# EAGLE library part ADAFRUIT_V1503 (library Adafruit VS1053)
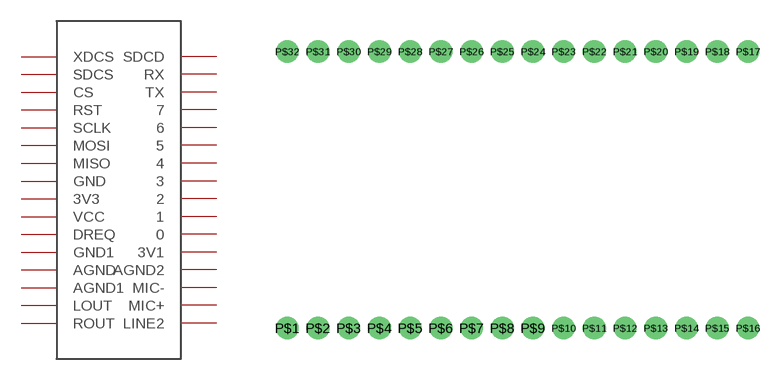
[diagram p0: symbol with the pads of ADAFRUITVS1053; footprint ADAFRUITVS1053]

Designator prefix -

## ADAFRUIT_V1503  [ADAFRUITVS1053]
P$1  XDCS
P$2  SDCS
P$3  CS
P$4  RST
P$5  SCLK
P$6  MOSI
P$7  MISO
P$8  GND
P$9  3V3
P$10  VCC
P$11  DREQ
P$12  GND1
P$13  AGND
P$14  AGND1
P$15  LOUT
P$16  ROUT
P$17  LINE2
P$18  MIC+
P$19  MIC-
P$20  AGND2
P$21  3V1
P$22  0
P$23  1
P$24  2
P$25  3
P$26  4
P$27  5
P$28  6
P$29  7
P$30  TX
P$31  RX
P$32  SDCD

## Footprint ADAFRUITVS1053 (pad centres in mm)
drill 1.016 pad 1.88: P$1 8.89,2.54; P$2 11.43,2.54; P$3 13.97,2.54; P$4 16.51,2.54; P$5 19.05,2.54; P$6 21.59,2.54; P$7 24.13,2.54; P$8 26.67,2.54; P$9 29.21,2.54; P$10 31.75,2.54; P$11 34.29,2.54; P$12 36.83,2.54; P$13 39.37,2.54; P$14 41.91,2.54; P$15 44.45,2.54; P$16 46.99,2.54; P$17 46.99,25.4; P$18 44.45,25.4; P$19 41.91,25.4; P$20 39.37,25.4; P$21 36.83,25.4; P$22 34.29,25.4; P$23 31.75,25.4; P$24 29.21,25.4; P$25 26.67,25.4; P$26 24.13,25.4; P$27 21.59,25.4; P$28 19.05,25.4; P$29 16.51,25.4; P$30 13.97,25.4; P$31 11.43,25.4; P$32 8.89,25.4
